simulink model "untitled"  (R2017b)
settings: Solver=ode15s  StartTime=0.0  StopTime=50  RelTol=1e-3
libraries: simulink x1

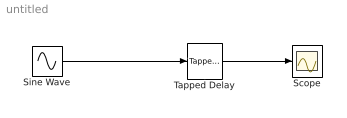
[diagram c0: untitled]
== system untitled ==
  Scope : Scope
  Sine Wave : Sin  SampleTime=0
  Tapped Delay : simulink/Discrete/Tapped Delay  vinit=0.0  samptime=1  NumDelays=3  DelayOrder=Oldest  includeCurrent=off
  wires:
  Sine Wave/1 -> Tapped Delay/1
  Tapped Delay/1 -> Scope/1
